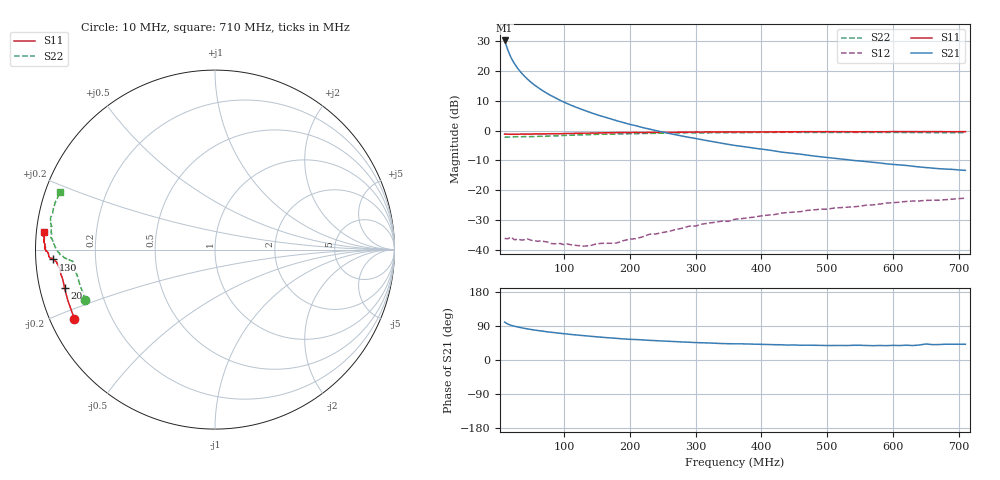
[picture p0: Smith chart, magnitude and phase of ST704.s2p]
!  POLYFET RF DEVICES
!  S PARAMETERS FOR
!  ST704
!  VDS=28, IDQ=800MA
! Date: Thu May 11 10:14:10 2000
# MHZ  S  MA  R  50.0000
! SCATTERING PARAMETERS :
! Freq=MHz Mag[s11] Ang[s11] Mag[s21] Ang[s21] Mag[s12] Ang[s12] Mag[s22] Ang[s22]
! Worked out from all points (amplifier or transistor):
!   81 points, 10 MHz to 710 MHz, reference 50 ohm
!   highest |S21| = 30.1 dB at 10 MHz (marker M1)
!   |S21| within 3 dB of that: start of sweep to 14.58 MHz
!   unconditionally stable (mu >= 1): 127.7 MHz to end of sweep
!   at 75 MHz: K = 0.55, MSG = 24.8 dB, |S12| = -37.3 dB
!   at 310 MHz: K = 1.06, MAG = 12.7 dB, |S12| = -31.3 dB
!   at 710 MHz: K = 1.20, MAG = 2.0 dB, |S12| = -22.6 dB
!   S11 on the Smith chart (normalised r, x): 10 MHz: 0.07, -0.23; 20 MHz: 0.07, -0.12; 130 MHz: 0.05, -0.03; 710 MHz: 0.02, +0.05
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10  0.8732 -153.8  32.01 100.1  0.01571 18.2  0.7747 -158.7
15  0.8676 -161.2  21.96 94.7  0.01551 9.1  0.7778 -165.3
20  0.8649 -165.8  16.31 91.4  0.01653 10.4  0.7805 -169.0
25  0.8641 -168.0  13.07 89.2  0.01487 5.2  0.7852 -170.7
30  0.8659 -169.9  10.89 87.1  0.01532 7.5  0.788 -172.2
35  0.8701 -170.7  9.305 85.3  0.01477 6.1  0.7855 -173.1
40  0.8692 -171.9  8.129 83.5  0.01493 5.5  0.7918 -173.8
45  0.8703 -172.7  7.176 82.1  0.01539 6.5  0.789 -174.2
50  0.8702 -173.0  6.418 80.5  0.01465 7.5  0.7903 -174.5
55  0.8766 -173.6  5.801 79.3  0.01448 7.0  0.7924 -174.7
65  0.8773 -174.2  4.859 76.8  0.01431 9.9  0.801 -175.6
80  0.8837 -175.0  3.856 73.3  0.01295 13.7  0.8105 -175.8
100  0.8893 -175.7  2.986 69.4  0.01236 18.8  0.826 -176.5
110  0.8928 -175.9  2.673 67.5  0.01234 24.2  0.8327 -176.6
130  0.9025 -176.5  2.195 64.3  0.01166 30.2  0.8476 -177.4
150  0.9081 -176.9  1.839 61.2  0.01278 41.2  0.8629 -178.1
180  0.9222 -177.2  1.461 57.1  0.01314 56.4  0.8756 -179.2
250  0.9312 -178.8  0.9421 50.1  0.01972 73.5  0.9026 176.9
360  0.95 179.1  0.5621 42.7  0.03296 84.1  0.9237 172.0
480  0.9541 177.3  0.3744 38.8  0.04712 85.1  0.9282 167.5
600  0.9604 175.5  0.2712 38.7  0.06216 87.6  0.9275 163.3
710  0.9581 174.0  0.2155 41.4  0.07397 89.1  0.9241 159.6
